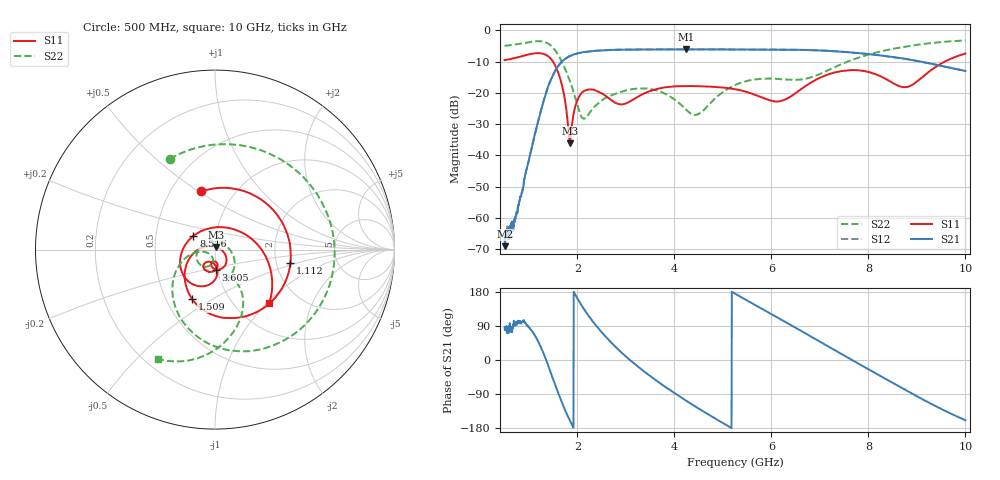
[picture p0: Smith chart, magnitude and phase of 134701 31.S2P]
!  2-Port S-parameters saved by WinCal
! VAR MeasName=S-Parameters (CALIBRATED_DATA) read from VNA (N5242A)
! VAR MeasDate=2013-7-3 16:33:16
! VAR NAME=134701 31
! VAR FILENAME=134701 31.S2P
! VAR DATE=2013-7-3 16:33:16
! VAR PHYS_PORTS=1,2
# Hz S MA R 50
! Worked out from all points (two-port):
!   1601 points, 500 MHz to 10 GHz, reference 50 ohm
!   highest |S21| = -6.11 dB at 4.235 GHz (marker M1); lowest = -69.0 dB at 505.9 MHz (marker M2)
!   |S21| within 3 dB of the highest: 1.752 GHz to 8.747 GHz (6.995 GHz wide, 133 % of centre)
!   lowest |S11| = -36.1 dB at 1.842 GHz (marker M3), VSWR 1.03, Z = 50.4 + j1.54 ohm
!   |S11| at or under -10 dB: 1.495 GHz to 9.578 GHz (8.083 GHz wide, 146 % of centre)
!   |S22| runs from -28.3 to -3.3 dB; largest |S21 - S12| = 0.0027
!   S11 on the Smith chart (normalised r, x): 500 MHz: 0.70, +0.51; 1.112 GHz: 2.39, -0.43; 1.509 GHz: 0.67, -0.41; 3.605 GHz: 0.98, -0.23; 8.516 GHz: 0.78, +0.12; 10 GHz: 1.43, -1.03
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5e8  0.3329 103.1  0.0004534 86.4  0.0005453 79.3  0.5645 116.5
5.059375e8  0.3335 102.1  0.0003565 78.7  0.0004741 91.7  0.565 115.7
7.01875e8  0.3585 69.4  0.0008643 92.9  0.0008764 100.8  0.5885 86.6
1.111562e9  0.4267 -10.0  0.01982 68.4  0.01989 68.0  0.6624 8.5
1.349062e9  0.4047 -68.3  0.09641 2.6  0.0966 2.5  0.6372 -51.6
1.509375e9  0.3036 -114.8  0.2001 -53.8  0.2 -54.0  0.5147 -96.6
1.6875e9  0.1276 -168.1  0.3181 -114.0  0.3178 -114.1  0.3056 -140.7
1.841875e9  0.01575 76.2  0.3857 -159.0  0.3856 -159.0  0.1571 -166.2
2.085312e9  0.09908 -51.9  0.4415 144.5  0.4417 144.4  0.04154 -149.4
2.429688e9  0.1045 -94.9  0.4723 84.0  0.4725 83.9  0.06788 -99.7
2.869062e9  0.06571 -95.8  0.4889 24.6  0.4885 24.5  0.102 -113.0
3.605312e9  0.1135 -88.3  0.4936 -52.3  0.4938 -52.3  0.1106 -158.2
3.670625e9  0.1168 -90.3  0.4943 -58.3  0.4936 -58.4  0.1071 -163.5
4.234688e9  0.1281 -106.5  0.4951 -106.8  0.4946 -106.7  0.05477 130.2
4.501875e9  0.1275 -112.1  0.4939 -128.1  0.4947 -128.2  0.04593 62.9
5.25e9  0.1145 -124.7  0.4925 175.2  0.4931 175.1  0.1331 -34.2
6.140625e9  0.07311 -105.7  0.4903 110.9  0.4907 110.9  0.1666 -70.6
6.835312e9  0.1487 -86.2  0.4811 60.5  0.4816 60.5  0.1787 -61.2
7.583438e9  0.2293 -122.6  0.445 5.8  0.4459 5.5  0.3177 -60.5
8.420625e9  0.157 162.2  0.3811 -54.6  0.3799 -54.8  0.4879 -79.9
8.515625e9  0.1423 147.8  0.3728 -61.3  0.3717 -61.5  0.5052 -82.2
1e10  0.424 -44.3  0.2237 -159.0  0.2233 -159.0  0.6861 -117.4
